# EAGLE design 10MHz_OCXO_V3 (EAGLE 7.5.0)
CNAME: 10MHz OXCO for PM6665/PM6669; CREVISION: V 0.2; DESIGNER: Jack Zimmermann
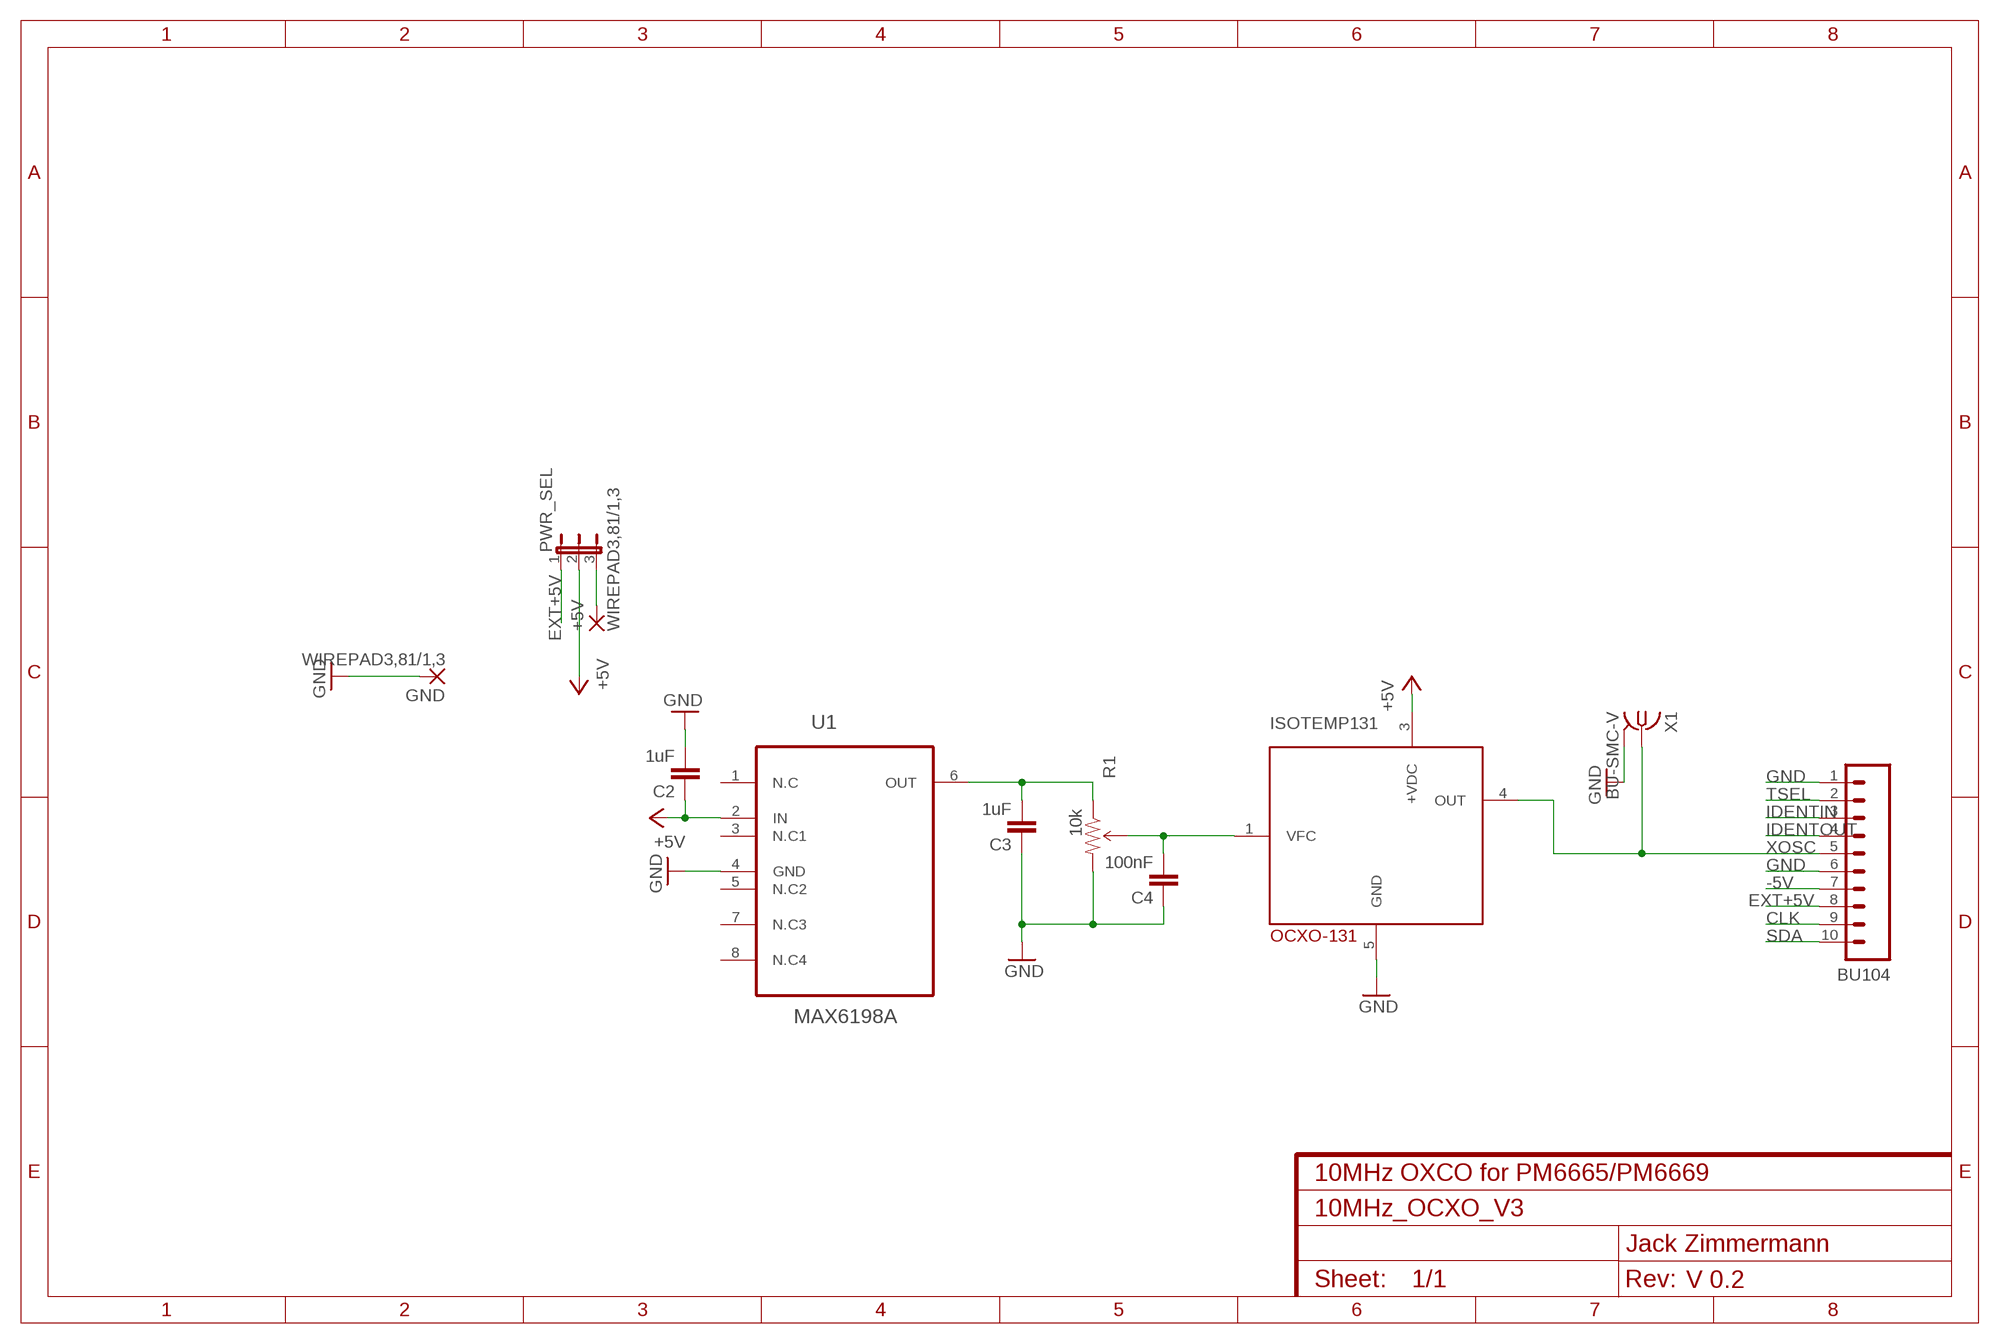
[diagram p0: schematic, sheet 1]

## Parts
+5V  WIREPAD3,81/1,3  [3,81/1,3]
BU104  M10SILK_FEMALE_PTH  [1X10]
C2  1uF  C5/5  [C5B5]
C3  1uF  C5/5  [C5B5]
C4  100nF  C5/2.5  [C5B2.5]
GND  WIREPAD3,81/1,3  [3,81/1,3]
ISOTEMP131  OCXO-131  [ISOTEMP131]
PWR_SEL  JP2E  [JP2]
R1  10k  TRIMPOT3362U-2  [3362U-2]
U1  MAX6198A  [SOIC127P600X175-8N]
X1  BU-SMC-V  [BU-SMC-V]

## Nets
+5V: C2.1 ISOTEMP131.3(+VDC) PWR_SEL.2 U1.2(IN)
-5V: BU104.7
CLK: BU104.9
EXT+5V: BU104.8 PWR_SEL.1
GND: BU104.1 BU104.6 C2.2 C3.1 C4.1 GND.1(P) ISOTEMP131.5(GND) R1.3(CW) U1.4(GND) X1.2 X1.3 X1.4 X1.5
IDENTIN: BU104.3
IDENTOUT: BU104.4
N$2: C3.2 R1.1(CCW) U1.6(OUT)
N$3: C4.2 ISOTEMP131.1(VFC) R1.2(WIPER)
N$4: +5V.1(P) PWR_SEL.3
SDA: BU104.10
TSEL: BU104.2
XOSC: BU104.5 ISOTEMP131.4(OUT) X1.1
Unconnected: U1.1(N.C) U1.3(N.C1) U1.5(N.C2) U1.7(N.C3) U1.8(N.C4)

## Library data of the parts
+5V GND = wirepad:WIREPAD: Wire PAD connect wire on PCB
BU104 = SparkFun-Connectors:M10: Header 10 Standard 10-pin 0.1" header. Use with straight break away headers (SKU : PRT-00116), right angle break away headers (PRT-00553), swiss pins (PRT-00743), machine pins (PRT-00117), and female headers (PRT-00115).; PROD_ID: CONN-11563
C2-C4 = capacitor-wima:C: CAPACITOR
ISOTEMP131 = jackens:OCXO-131
PWR_SEL = jumper:JP2E: JUMPER
R1 = SparkFun-Electromechanical:TRIMPOT: Various small potentiometers for "set-and-forget" applications
U1 = jackens:MAX6198A: MAX6198A Precision, Micropower, Low-Dropout Voltage Reference Output voltage 4.096V ±2mV; MPN: MAX6198A; PACKAGE: SOIC-8; RS-ONLINE: 732-9743; SUPPLIER: Maxim
X1 = con-coax:BU-SMC-V: FEMALE SMC CONNECTOR; OC_FARNELL: unknown; OC_NEWARK: unknown

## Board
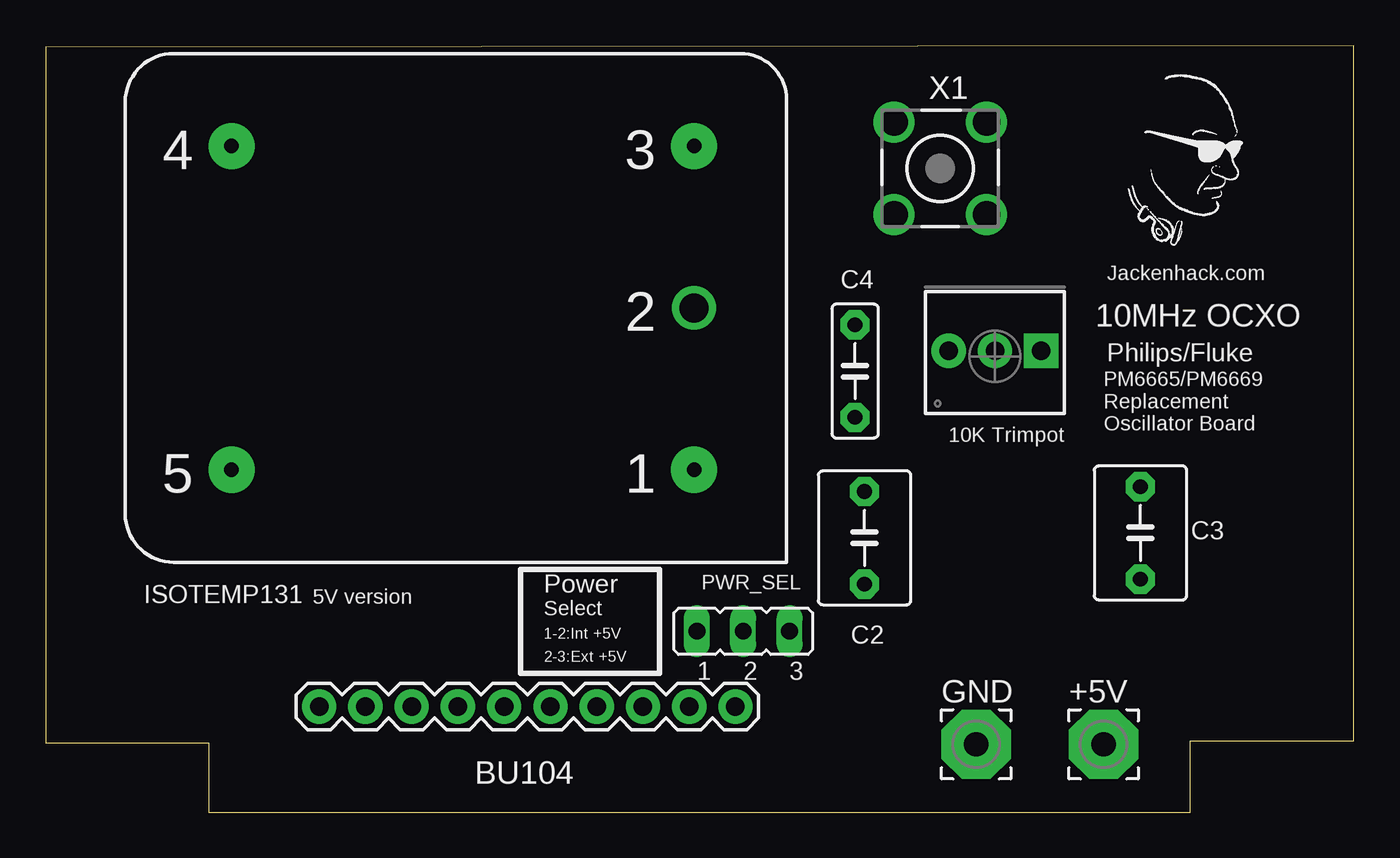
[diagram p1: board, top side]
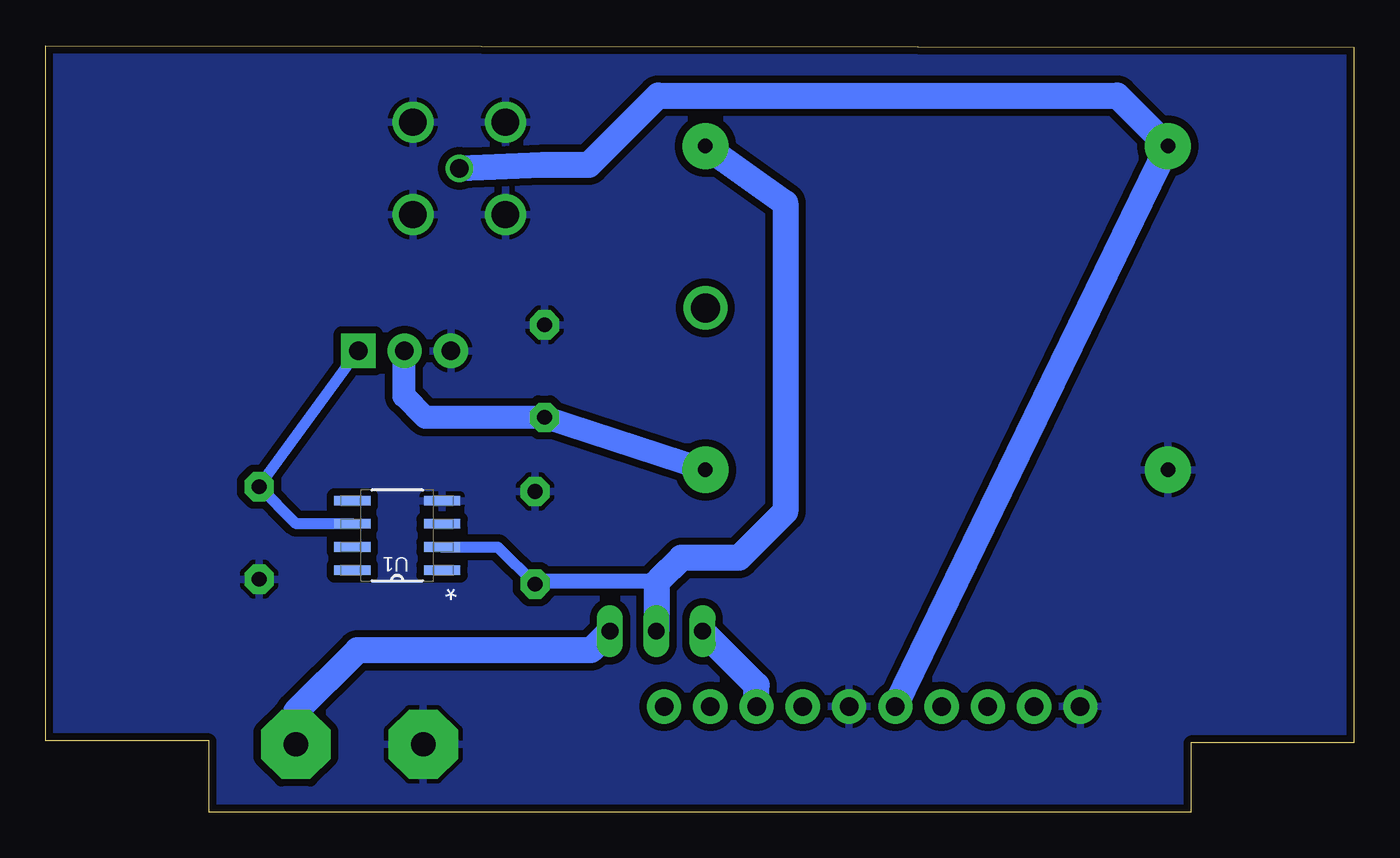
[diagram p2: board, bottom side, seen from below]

Size 71.86 x 42.12 mm. Coordinates in mm from the lower left corner, seen from the top.
Outline: 8.95,0 62.88,0 62.88,3.91 71.86,3.91 71.86,42.12 0,42.02 0,3.81 8.95,3.81 8.95,0
Copper layers (1*16): Top 0.035mm / dielectric 1.5mm / Bottom 0.035mm
Design rules "dirt_cheap_dirty_boards.v1": minimum track width 5mil, minimum drill 12mil, track to track 5mil, track to pad 5mil, pad to pad 5mil, via to via 5mil, smd to smd 0mil, copper to edge 10mil, drill to drill 10mil, minimum pad ring 10mil, minimum via ring 6mil, stop-mask expansion 2mil, vias tented up to drill 25mil, thermal gap 10mil

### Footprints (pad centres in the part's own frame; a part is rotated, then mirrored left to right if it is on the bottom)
3,81/1,3 = drill 1.321 pad 3.81 octagon: 1 0,0
1X10 = drill 1.016 pad 1.88: 1 0,0; 2 2.54,0; 3 5.08,0; 4 7.62,0; 5 10.16,0; 6 12.7,0; 7 15.24,0; 8 17.78,0; 9 20.32,0; 10 22.86,0
C5B5 = drill 0.813 pad 1.6 octagon: 1 -2.54,0; 2 2.54,0
C5B2.5 = drill 0.813 pad 1.6 octagon: 1 -2.54,0; 2 2.54,0
ISOTEMP131 = drill 0.8 pad 2.54: 1 -5.08,-10.16; 3 -5.08,7.62; 4 -30.48,7.62; 5 -30.48,-10.16 | drill 1.6 pad 2.184: 2 -5.08,-1.27
JP2 = drill 0.914 long: 1 -2.54,0; 2 0,0; 3 2.54,0
3362U-2 = drill 1.016 pad 1.88 square: 1 -2.54,-0.305 | drill 1.016 pad 1.88: 2 0,-0.305; 3 2.54,-0.305
SOIC127P600X175-8N = smd 1.981 x 0.533: 1 -2.464,1.905; 2 -2.464,0.635; 3 -2.464,-0.635; 4 -2.464,-1.905; 5 2.464,-1.905; 6 2.464,-0.635; 7 2.464,0.635; 8 2.464,1.905
BU-SMC-V = drill 1.016: 1 0,0 | drill 1.5: 2 -2.54,2.54; 3 2.54,2.54; 4 2.54,-2.54; 5 -2.54,-2.54

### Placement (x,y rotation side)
+5V  58.11,3.73 0 top
BU104  15.03,5.8 0 top
C2  44.98,15.07 90 top
C3  60.13,15.34 90 top
C4  44.46,24.23 270 top
GND  51.11,3.73 0 top
ISOTEMP131  40.7,28.97 0 top
PWR_SEL  38.32,9.94 0 top
R1  52.14,25.04 180 top
U1  52.55,15.21 180 bottom
X1  49.14,35.37 0 top

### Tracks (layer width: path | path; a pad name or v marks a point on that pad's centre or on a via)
+5V
  Bottom 0.61: U1.2 47.02,14.57 C2.1
  Bottom 0.813: C2.1 44.81,12.7 38.21,12.7
  Bottom 1.422: ISOTEMP131.3 31.23,33.47 31.23,16.51 33.77,13.97 36.94,13.97 38.21,12.7 38.32,12.59 PWR_SEL.2
EXT+5V
  Bottom 1.422: BU104.8 32.81,6.97 PWR_SEL.1
GND
  pour Bottom (isolate 0.406): -0.4,43.65 72.46,43.65 72.46,0.27 -0.4,-1
N$2
  Bottom 0.61: U1.6 58.09,15.84 C3.2 R1.1
N$3
  Bottom 1.27: ISOTEMP131.1 C4.2 51.01,21.69 52.18,22.86 52.18,25.3 R1.2
N$4
  Bottom 1.422: PWR_SEL.3 41.9,8.89 54.72,8.89 58.11,5.5 +5V.1
XOSC
  Bottom 1.422: BU104.5 ISOTEMP131.4 13,39.37 38.21,39.37 42.02,35.56 44.56,35.56 X1.1

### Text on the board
tPlace: Philips/Fluke | PM6665/PM6669 / Replacement / Oscillator Board
tNames: Jackenhack.com | 10MHz OCXO | 10K Trimpot | Power | 5V version | Select | 1-2:Int +5V | 2-3:Ext +5V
